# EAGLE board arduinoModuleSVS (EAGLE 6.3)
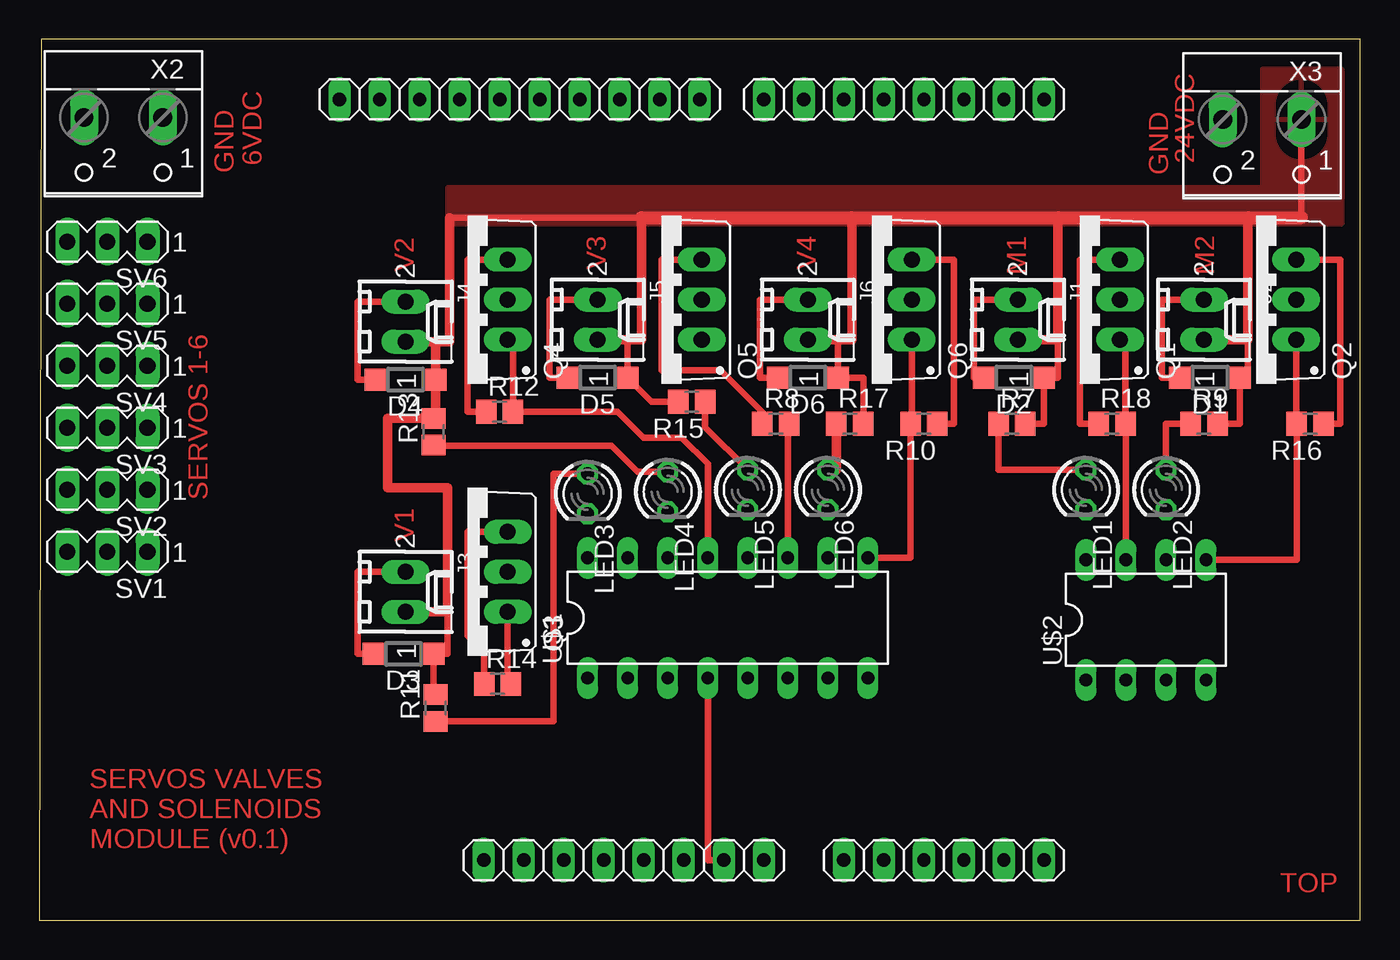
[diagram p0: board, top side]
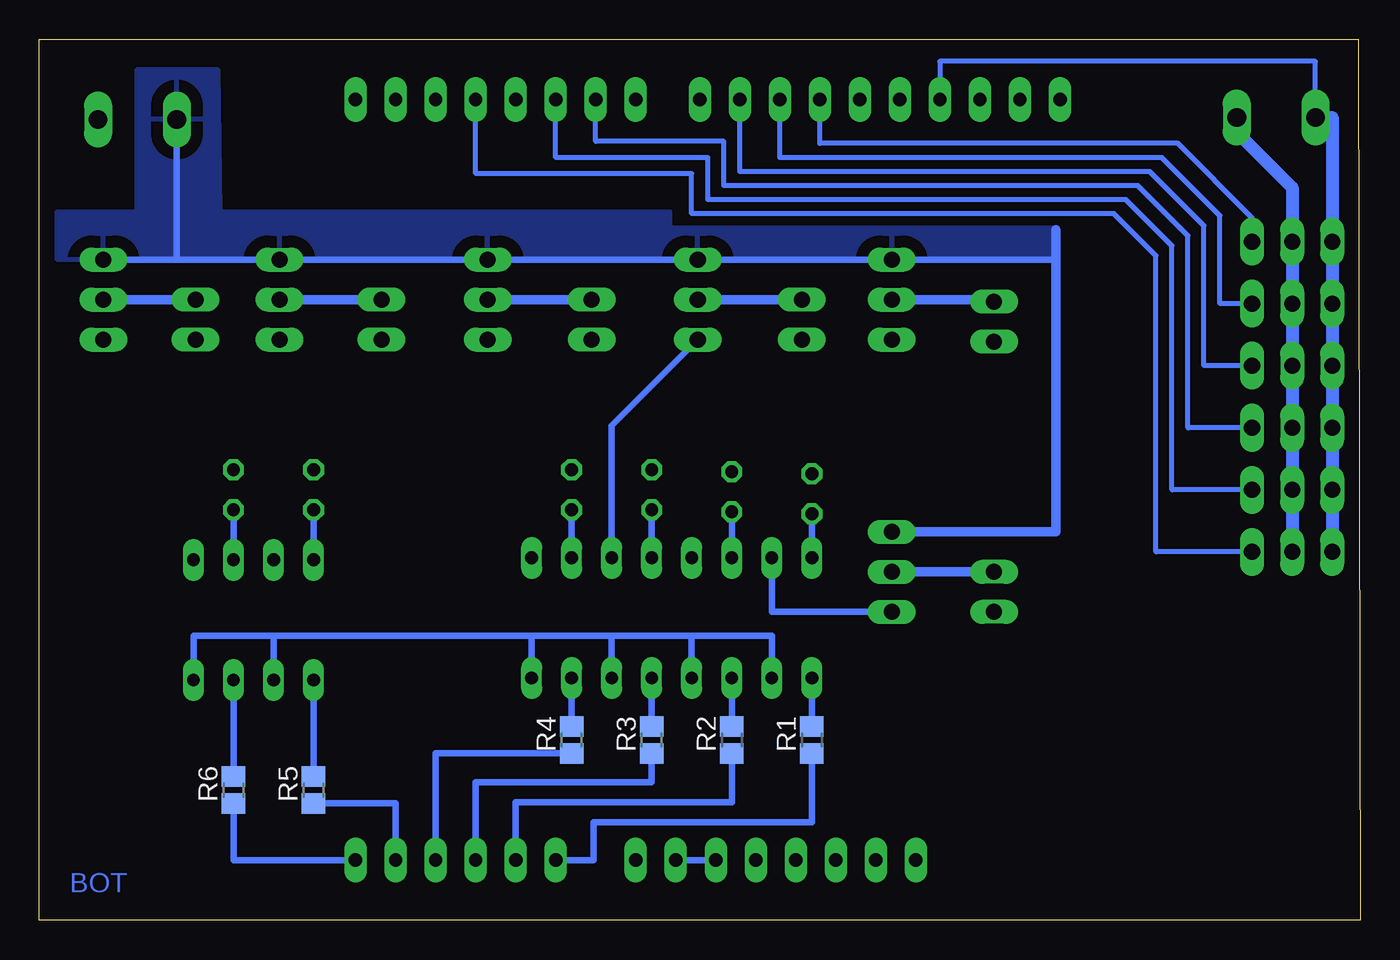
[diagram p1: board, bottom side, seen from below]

Size 83.82 x 55.88 mm. Coordinates in mm from the lower left corner, seen from the top.
Outline: 83.82,0 83.82,55.88 0.13,55.88 0,0 83.82,0
Copper layers (1*16): Top 0.035mm / dielectric 1.5mm / Bottom 0.035mm
Design rules "default *": minimum track width 10mil, minimum drill 22mil, track to track 0.5mm, track to pad 0.5mm, pad to pad 0.5mm, via to via 0.5mm, smd to smd 0.5mm, copper to edge 26mil, drill to drill 8mil, minimum pad ring 10mil, minimum via ring 10mil, stop-mask expansion 4mil, vias tented up to drill 0mil, thermal gap 30mil
Net classes: 1 power: width 0.61 mm, drill 0.61 mm, clearance 0.254 mm; 2 gnd: width 0.305 mm, drill 0.559 mm, clearance 0.254 mm; 3 usbvcc: width 0.508 mm, drill 0.61 mm, clearance 0.254 mm; 4 aref: width 0.406 mm, drill 0.61 mm, clearance 0.254 mm

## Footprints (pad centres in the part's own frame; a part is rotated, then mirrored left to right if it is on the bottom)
1X06 = drill 0.85 pad 1.422 long: 1 -6.35,0; 2 -3.81,0; 3 -1.27,0; 4 1.27,0; 5 3.81,0; 6 6.35,0
SOD123 = smd 1.4 x 1.4: A 1.9,0; C -1.9,0
1X10@1 = drill 0.85 pad 1.422 long: 1 -11.43,0; 2 -8.89,0; 3 -6.35,0; 4 -3.81,0; 5 -1.27,0; 6 1.27,0; 7 3.81,0; 8 6.35,0; 9 8.89,0; 10 11.43,0
1X08 = drill 0.85 pad 1.422 long: 1 -8.89,0; 2 -6.35,0; 3 -3.81,0; 4 -1.27,0; 5 1.27,0; 6 3.81,0; 7 6.35,0; 8 8.89,0
6410-02 = drill 1.016 long: 1 1.27,0; 2 -1.27,0
LED3MM = drill 0.813 octagon: A -1.27,0; K 1.27,0
TO220BV = drill 1.016 long: D 0,-2.54; G -2.54,-2.54; S 2.54,-2.54
R0805 = smd 1.3 x 1.5: 1 -0.85,0; 2 0.85,0
MA03-1 = drill 1.016 long: 1 -2.54,0; 2 0,0; 3 2.54,0
DIL16 = drill 0.813 long: 1 -8.89,-3.81; 2 -6.35,-3.81; 3 -3.81,-3.81; 4 -1.27,-3.81; 5 1.27,-3.81; 6 3.81,-3.81; 7 6.35,-3.81; 8 8.89,-3.81; 9 8.89,3.81; 10 6.35,3.81; 11 3.81,3.81; 12 1.27,3.81; 13 -1.27,3.81; 14 -3.81,3.81; 15 -6.35,3.81; 16 -8.89,3.81
DIL08 = drill 0.813 long: 1 -3.81,-3.81; 2 -1.27,-3.81; 3 1.27,-3.81; 4 3.81,-3.81; 5 3.81,3.81; 6 1.27,3.81; 7 -1.27,3.81; 8 -3.81,3.81
W237-102 = drill 1.194 long: 1 -2.5,-1.27; 2 2.5,-1.27

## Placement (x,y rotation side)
AD  6x1F-H8.5  [1X06]  57.4,3.81 0 top
D1  [SOD123]  74.3,34.42 180 top
D2  [SOD123]  61.85,34.42 180 top
D3  [SOD123]  23.11,16.89 180 top
D4  [SOD123]  23.24,34.29 180 top
D5  [SOD123]  35.43,34.42 180 top
D6  [SOD123]  48.77,34.42 180 top
IOH  10x1F-H8.5  [1X10@1]  30.48,52.07 180 top
IOL  8x1F-H8.5  [1X08]  54.86,52.07 180 top
J1  22-27-2021-02  [6410-02]  62.1,38.1 270 top
J2  22-27-2021-02  [6410-02]  73.91,38.1 270 top
J3  22-27-2021-02  [6410-02]  23.24,20.83 270 top
J4  22-27-2021-02  [6410-02]  23.24,37.97 270 top
J5  22-27-2021-02  [6410-02]  35.43,38.1 270 top
J6  22-27-2021-02  [6410-02]  48.77,38.1 270 top
LED1  [LED3MM]  66.42,27.3 270 top
LED2  [LED3MM]  71.5,27.3 270 top
LED3  [LED3MM]  34.8,27.05 270 top
LED4  [LED3MM]  39.88,27.18 270 top
LED5  [LED3MM]  44.96,27.3 270 top
LED6  [LED3MM]  50.04,27.3 270 top
POWER  8x1F-H8.5  [1X08]  37.08,3.81 0 top
Q1  IRF512  [TO220BV]  66.04,39.37 90 top
Q2  IRF512  [TO220BV]  77.22,39.37 90 top
Q3  IRF512  [TO220BV]  27.18,22.1 90 top
Q4  IRF512  [TO220BV]  27.18,39.37 90 top
Q5  IRF512  [TO220BV]  39.5,39.37 90 top
Q6  IRF512  [TO220BV]  52.83,39.37 90 top
R1  [R0805]  34.8,11.43 90 bottom
R2  [R0805]  39.88,11.43 90 bottom
R3  [R0805]  44.96,11.43 90 bottom
R4  [R0805]  50.04,11.43 90 bottom
R5  [R0805]  66.42,8.26 90 bottom
R6  [R0805]  71.5,8.26 90 bottom
R7  1K  [R0805]  61.72,31.5 0 top
R8  1K  [R0805]  46.74,31.5 0 top
R9  1K  [R0805]  73.91,31.5 0 top
R10  1K  [R0805]  56.13,31.5 180 top
R11  1K  [R0805]  25.15,13.46 90 top
R12  1K  [R0805]  29.21,32.26 0 top
R13  1K  [R0805]  25.02,30.99 90 top
R14  1K  [R0805]  29.08,14.99 0 top
R15  1K  [R0805]  41.4,32.89 180 top
R16  1K  [R0805]  80.65,31.5 180 top
R17  1K  [R0805]  51.43,31.5 0 top
R18  1K  [R0805]  68.07,31.5 0 top
SV1  [MA03-1]  4.32,23.37 180 top
SV2  [MA03-1]  4.32,27.3 180 top
SV3  [MA03-1]  4.32,31.24 180 top
SV4  [MA03-1]  4.32,35.18 180 top
SV5  [MA03-1]  4.32,39.12 180 top
SV6  [MA03-1]  4.32,43.05 180 top
U$1  ACPL-847-W00E  [DIL16]  43.69,19.18 0 top
U$2  ACPL-827-00CE  [DIL08]  70.23,19.05 0 top
X2  [W237-102]  5.33,49.66 180 top
X3  [W237-102]  77.6,49.53 180 top

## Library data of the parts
AD IOH IOL POWER = SmartPrj
D1-D6 = diode
J1-J6 = con-molex; OC_FARNELL: unknown; OC_NEWARK: unknown
LED1-LED6 = led
Q1-Q6 = transistor-power
R1-R18 = resistor
SV1-SV6 = con-lstb; OC_FARNELL: unknown; OC_NEWARK: unknown
U$1 U$2 = wingX
X2 X3 = con-wago-500; MPN: 237-102; OC_FARNELL: unknown; OC_NEWARK: 70K9898

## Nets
GND: POWER.6 POWER.7 U$1.2 U$1.4 U$1.6 U$1.8 U$2.2 U$2.4
GND24V: Q1.S Q2.S Q3.S Q4.S Q5.S Q6.S R8.1 R10.1 R12.1 R14.1 R16.1 R18.1 X3.2
GNDARDUINO: IOH.7 SV1.3 SV2.3 SV3.3 SV4.3 SV5.3 SV6.3 X2.2
N$1: IOL.4 SV1.1
N$2: IOL.6 SV2.1
N$3: IOL.7 SV3.1
N$4: IOH.2 SV4.1
N$5: IOH.3 SV5.1
N$6: IOH.4 SV6.1
N$7: R1.2 U$1.1
N$8: R2.2 U$1.3
N$9: R3.2 U$1.5
N$10: AD.1 R1.1
N$11: R4.2 U$1.7
N$12: AD.2 R2.1
N$13: AD.3 R3.1
N$14: AD.4 R4.1
N$15: R6.2 U$2.3
N$16: R5.2 U$2.1
N$17: AD.6 R6.1
N$18: AD.5 R5.1
N$19: Q1.G R18.2 U$2.7
N$20: D2.A J1.2 Q1.D
N$21: LED2.K U$2.6
N$22: LED2.A R9.1
N$23: Q2.G R16.2 U$2.5
N$24: LED1.K U$2.8
N$25: D1.A J2.2 Q2.D
N$26: LED1.A R7.1
N$27: LED3.K U$1.16
N$28: LED3.A R11.1
N$29: Q3.G R14.2 U$1.15
N$30: D3.A J3.2 Q3.D
N$31: LED4.K U$1.14
N$32: LED4.A R13.1
N$33: Q4.G R12.2 U$1.13
N$34: D4.A J4.2 Q4.D
N$35: LED5.K U$1.12
N$36: LED5.A R15.1
N$37: Q5.G R8.2 U$1.11
N$38: D5.A J5.2 Q5.D
N$39: LED6.K U$1.10
N$40: LED6.A R17.1
N$41: Q6.G R10.2 U$1.9
N$42: D6.A J6.2 Q6.D
VCC6V: SV1.2 SV2.2 SV3.2 SV4.2 SV5.2 SV6.2 X2.1
VCC24: D1.C D2.C D3.C D4.C D5.C D6.C J1.1 J2.1 J3.1 J4.1 J5.1 J6.1 R7.2 R9.2 R11.2 R13.2 R15.2 R17.2 X3.1

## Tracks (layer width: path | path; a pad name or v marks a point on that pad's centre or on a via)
GND
  Top 0.406: POWER.7 42.42,3.81 U$1.4
  Bottom 0.406: POWER.6 POWER.7 | U$2.4 74.04,18.03 68.96,18.03 | 68.96,18.03 U$2.2 | U$1.2 37.34,18.03 42.42,18.03 | 47.5,18.03 42.8,18.03 42.42,18.03 | 47.5,18.03 52.58,18.03 | 52.58,18.03 68.96,18.03 | U$1.8 52.58,18.03 | U$1.6 47.5,18.03 | U$1.4 42.42,18.03
GND24V
  Top 0.406: Q2.S 82.55,41.91 82.55,31.5 R16.1 | Q1.S 66.04,41.91 66.04,31.5 R18.1 | Q5.S 39.5,41.91 39.5,34.89 43.22,34.89 45.89,32.22 R8.1 | Q4.S 27.18,41.91 27.18,32.26 R12.1 | R14.1 28.23,16.98 27.18,18.03 27.18,24.64 Q3.S | R10.1 58.04,31.5 58.04,41.91 Q6.S
  Bottom 0.406: 75.1,41.91 Q1.S Q6.S Q5.S Q4.S 19.3,41.91 | 75.1,41.91 Q2.S | X3.2 75.1,41.91
  Bottom 0.61: Q3.S 19.3,24.64 19.3,41.91 19.3,43.82
  pour Bottom: 19.3,41.91 82.68,41.91 82.68,44.96 77.6,44.96 77.6,53.98 72.52,53.98 72.39,44.96 43.81,44.96 43.81,43.94 19.3,43.94
GNDARDUINO
  Bottom 0.305: X2.2 2.83,54.48 26.67,54.48 IOH.7
  Bottom 0.813: X2.2 1.78,50.93 SV6.3 SV5.3 SV4.3 SV3.3 SV2.3 SV1.3
N$1
  Bottom 0.305: SV1.1 12.95,23.37 12.95,42.16 15.62,44.83 42.42,44.83 42.42,47.37 56.13,47.37 IOL.4
N$2
  Bottom 0.305: SV2.1 11.94,27.3 11.94,42.8 14.86,45.72 41.4,45.72 41.4,48.39 51.05,48.39 IOL.6
N$3
  Bottom 0.305: SV3.1 10.92,31.24 10.92,43.43 14.1,46.61 40.39,46.61 40.39,49.4 48.51,49.4 IOL.7
N$4
  Bottom 0.305: SV4.1 9.91,35.18 9.91,44.07 13.33,47.5 39.37,47.5 IOH.2
N$5
  Bottom 0.305: SV5.1 8.89,39.12 8.89,44.7 12.57,48.39 36.83,48.39 IOH.3
N$6
  Bottom 0.305: SV6.1 6.86,44.58 11.56,49.28 34.29,49.28 IOH.4
N$7
  Bottom 0.406: R1.2 U$1.1
N$8
  Bottom 0.406: R2.2 U$1.3
N$9
  Bottom 0.406: R3.2 U$1.5
N$10
  Bottom 0.406: AD.1 48.64,3.81 48.64,6.22 34.8,6.22 R1.1
N$11
  Bottom 0.406: R4.2 U$1.7
N$12
  Bottom 0.406: AD.2 53.59,7.49 39.88,7.49 R2.1
N$13
  Bottom 0.406: AD.3 56.13,8.76 44.96,8.76 R3.1
N$14
  Bottom 0.406: AD.4 58.67,10.58 R4.1
N$15
  Bottom 0.406: R6.2 U$2.3
N$16
  Bottom 0.406: R5.2 U$2.1
N$17
  Bottom 0.406: AD.6 71.5,3.81 R6.1
N$18
  Bottom 0.406: AD.5 61.21,7.4 R5.1
N$19
  Top 0.406: U$2.7 68.96,31.5 R18.2 68.92,36.83 Q1.G
N$20
  Top 0.406: D2.A 59.31,34.42 59.31,39.37 J1.2
  Bottom 0.61: J1.2 Q1.D
N$21
  Bottom 0.406: LED2.K U$2.6
N$22
  Top 0.406: R9.1 71.5,31.5 LED2.A
N$23
  Top 0.406: Q2.G 79.76,31.5 R16.2 79.8,22.86 U$2.5
N$24
  Bottom 0.406: LED1.K U$2.8
N$25
  Top 0.406: D1.A 71.25,34.42 71.25,39.37 J2.2
  Bottom 0.61: J2.2 Q2.D
N$26
  Top 0.406: R7.1 60.87,28.57 LED1.A
N$27
  Bottom 0.406: U$1.16 LED3.K
N$28
  Top 0.406: R11.1 32.64,12.61 32.64,28.32 LED3.A
N$29
  Top 0.406: R14.2 29.72,14.99 Q3.G
  Bottom 0.406: Q3.G 37.34,19.56 U$1.15
N$30
  Top 0.406: D3.A 20.19,16.89 20.19,22.1 J3.2
  Bottom 0.61: J3.2 Q3.D
N$31
  Bottom 0.406: U$1.14 LED4.K
N$32
  Top 0.406: R13.1 25.02,30.1 36.32,30.1 37.97,28.45 LED4.A
N$33
  Top 0.406: Q4.G 30.06,36.83 R12.2 36.7,32.26 38.35,30.61 40.77,30.61 42.42,28.96 U$1.13
N$34
  Top 0.406: D4.A 20.19,34.29 20.19,39.24 J4.2
  Bottom 0.406: J4.2 23.24,39.37
  Bottom 0.61: 23.24,39.37 Q4.D
N$35
  Bottom 0.406: U$1.12 LED5.K
N$36
  Top 0.406: R15.1 42.25,31.28 LED5.A
N$37
  Top 0.406: R8.2 47.5,31.41 U$1.11
  Bottom 0.406: Q5.G 47.5,31.37 U$1.11
N$38
  Top 0.406: D5.A 32.38,34.42 32.38,39.37 J5.2
  Bottom 0.61: Q5.D J5.2
N$39
  Bottom 0.406: U$1.10 LED6.K
N$40
  Top 0.61: R17.1 50.59,28.57 LED6.A
N$41
  Top 0.406: Q6.G 55.37,31.5 R10.2 55.28,22.99 U$1.9
N$42
  Top 0.406: D6.A 45.72,34.42 45.72,39.37 J6.2
  Bottom 0.61: J6.2 Q6.D
VCC6V
  Bottom 0.813: X2.1 7.83,50 4.32,46.48 SV6.2 SV5.2 SV4.2 SV3.2 SV2.2 SV1.2
VCC24
  Top 0.406: 80.1,44.58 X3.1 | 50.67,36.83 D6.C 52.28,34.42 R17.2 | J5.1 37.33,36.83 D5.C 38.86,32.89 R15.2 | 26.04,44.58 38.23,44.58 | 25.14,31.96 R13.2 | R11.2 25.01,14.31 D3.C 25.91,16.89 25.91,19.56 | R7.2 63.75,31.5 D2.C 64.64,34.42 64.64,36.83 | 76.71,36.83 76.71,34.93 arc-90 D1.C 76.2,31.5 R9.2
  Top 0.61: J2.1 76.71,36.83 76.71,44.58 | J1.1 64.64,36.83 64.64,44.58 | J6.1 50.67,36.83 51.56,36.83 51.56,44.58 | J5.1 38.23,36.83 38.23,44.58 | 25.14,36.7 D4.C 25.14,31.96 | 25.14,36.7 J4.1 | 25.14,36.7 26.04,36.7 26.04,44.58 | J3.1 25.91,19.56 25.91,27.43 22.1,27.43 22.1,31.84 R13.2
  Top 0.813: 80.1,44.58 76.71,44.58 64.64,44.58 51.56,44.58 38.23,44.58
  pour Top: 77.6,53.98 77.6,46.48 25.91,46.48 25.91,44.2 82.68,44.2 82.68,53.98

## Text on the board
Top: 24VDC | GND | GND | 6VDC | V2 | V3 | V4 | M1 | M2 | SERVOS 1-6 | V1 | SERVOS VALVES / AND SOLENOIDS / MODULE (v0.1) | TOP
Bottom: BOT
214bmp: D:/SmartProjects/Snc/a4_bn_logo2.bmp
